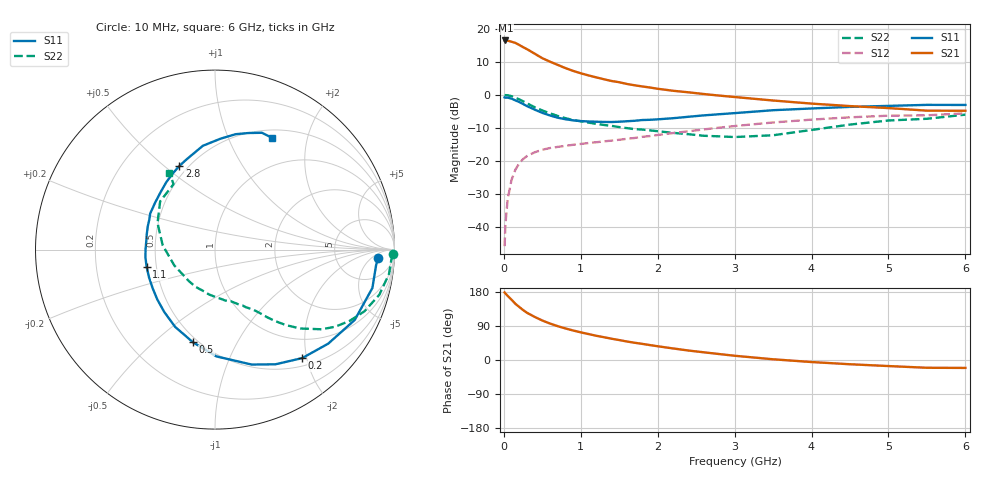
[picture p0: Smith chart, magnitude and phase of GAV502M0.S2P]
! Infineon Technologies  Discrete & RF Semiconductors
! BF775
! Si NPN RF Bipolar Junction Transistor in SOT23
! VCE = 0.5 V  IC = 2 mA
! Common Emitter S-Parameters:  May  1996
# GHz  S  MA  R  50
!  f  S11  S21  S12  S22
! GHz  MAG  ANG  MAG  ANG  MAG  ANG  MAG  ANG
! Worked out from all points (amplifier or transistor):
!   36 points, 10 MHz to 6 GHz, reference 50 ohm
!   highest |S21| = 16.4 dB at 20 MHz (marker M1)
!   |S21| within 3 dB of that: start of sweep to 327.4 MHz
!   unconditionally stable (mu >= 1): 996 MHz to end of sweep
!   at 250 MHz: K = 0.31, MSG = 16.9 dB, |S12| = -19.5 dB
!   at 1.4 GHz: K = 1.20, MAG = 6.3 dB, |S12| = -13.9 dB
!   at 6 GHz: K = 1.10, MAG = -1.5 dB, |S12| = -5.6 dB
!   S11 on the Smith chart (normalised r, x): 10 MHz: 17, -9; 200 MHz: 0.63, -1.92; 500 MHz: 0.47, -0.68; 1.1 GHz: 0.44, -0.10; 2.8 GHz: 0.45, +0.56; 6 GHz: 0.60, +1.46
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0.01  0.9101 -2.8  6.527 178.2  0.0051 88.4  0.9926 -1.5
0.02  0.9016 -5.6  6.615 175.6  0.0106 86.3  0.9842 -3.2
0.05  0.9026 -13.7  6.56 169.2  0.0264 81.6  0.9793 -7.9
0.1  0.8717 -26.7  6.325 159.2  0.0513 74.2  0.9494 -15.4
0.15  0.8201 -39.7  6.073 148.3  0.0731 66.6  0.901 -22.4
0.2  0.7756 -51.2  5.651 140.0  0.0913 60.9  0.8488 -27.9
0.25  0.7224 -62.2  5.247 131.9  0.1061 55.5  0.7957 -32.7
0.3  0.6723 -72.3  4.888 124.7  0.1177 51.6  0.7411 -36.8
0.4  0.5953 -89.2  4.18 113.8  0.1343 45.2  0.6469 -42.8
0.5  0.5311 -103.3  3.564 104.2  0.1468 40.7  0.5768 -46.8
0.6  0.4848 -117.2  3.159 96.2  0.1559 37.9  0.5226 -49.8
0.7  0.4481 -129.1  2.825 89.3  0.162 36.1  0.4771 -52.3
0.9  0.4089 -148.0  2.292 77.9  0.1743 34.5  0.4138 -56.1
1.1  0.393 -165.8  1.957 68.5  0.1856 33.6  0.3779 -59.9
1.4  0.3858 172.8  1.611 56.2  0.202 33.4  0.3373 -66.1
1.6  0.3963 160.9  1.453 48.8  0.2149 34.1  0.312 -70.6
2.2  0.4404 133.6  1.146 30.5  0.2626 33.9  0.2644 -89.2
2.8  0.506 113.2  0.969 15.7  0.3166 30.6  0.2341 -117.1
3.5  0.5822 96.7  0.816 1.9  0.3795 23.8  0.2433 -158.8
4.5  0.6535 79.8  0.672 -11.2  0.4543 12.0  0.3529 155.2
5.5  0.7014 68.1  0.573 -20.5  0.4878 -1.2  0.4318 122.3
6  0.6989 62.9  0.571 -20.9  0.5224 -4.7  0.4986 120.8
